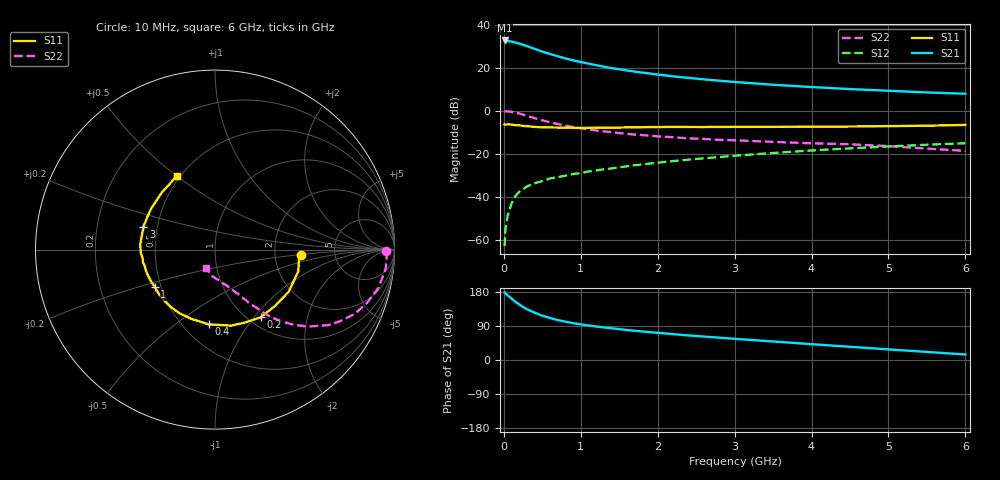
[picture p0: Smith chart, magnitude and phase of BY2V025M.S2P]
! SIEMENS Small Signal Semiconductors
! BFY420
! Si NPN RF SIEGET Grounded Emitter Transistor in MICRO-X
! VCE = 2 V  IC = 25 mA
! Common Emitter S-Parameters:  October  1996
# GHz  S  MA  R  50
!  f  S11  S21  S12  S22
! GHz  MAG  ANG  MAG  ANG  MAG  ANG  MAG  ANG
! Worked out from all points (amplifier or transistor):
!   36 points, 10 MHz to 6 GHz, reference 50 ohm
!   highest |S21| = 32.6 dB at 10 MHz (marker M1)
!   |S21| within 3 dB of that: start of sweep to 327.9 MHz
!   unconditionally stable (mu >= 1): start of sweep to 10.06 MHz; 1.732 GHz to end of sweep
!   at 250 MHz: K = 0.33, MSG = 33.6 dB, |S12| = -36.6 dB
!   at 1.4 GHz: K = 0.95, MSG = 23.4 dB, |S12| = -26.9 dB
!   at 6 GHz: K = 1.07, MAG = 9.9 dB, |S12| = -15.2 dB
!   S11 on the Smith chart (normalised r, x): 10 MHz: 2.82, -0.21; 200 MHz: 1.14, -1.08; 400 MHz: 0.66, -0.67; 1 GHz: 0.46, -0.23; 3 GHz: 0.42, +0.13; 6 GHz: 0.48, +0.50
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0.01  0.4791 -3.4  42.9 178.6  0.0007 119.4  0.9507 -0.5
0.02  0.4714 -6.6  42.76 175.4  0.0017 85.4  0.9582 -2.0
0.1  0.473 -29.8  40.4 162.4  0.0069 79.2  0.9355 -13.2
0.15  0.4587 -43.3  38.34 153.5  0.0102 74.1  0.8978 -19.3
0.2  0.4553 -56.0  36.35 146.8  0.0129 71.5  0.8571 -24.7
0.25  0.4396 -67.4  33.93 139.8  0.0148 67.5  0.8053 -29.6
0.3  0.4334 -77.9  31.62 134.1  0.0172 65.9  0.7588 -33.7
0.4  0.4178 -94.9  27.37 125.0  0.0203 62.6  0.6688 -39.9
0.5  0.4078 -109.0  23.56 116.9  0.023 59.9  0.5955 -44.3
0.6  0.4063 -120.0  20.78 110.9  0.0263 59.4  0.5357 -47.7
0.7  0.4032 -128.8  18.44 105.5  0.0283 59.2  0.4879 -50.4
0.8  0.4012 -136.5  16.4 101.1  0.0305 58.5  0.4471 -52.3
1  0.3944 -148.2  13.47 94.1  0.0352 59.0  0.3893 -55.0
1.1  0.3974 -153.1  12.39 91.2  0.0382 59.4  0.3663 -56.7
1.3  0.4014 -160.9  10.52 85.9  0.0432 59.2  0.3286 -58.6
1.6  0.4079 -170.3  8.589 79.2  0.0505 59.0  0.2876 -61.8
2.2  0.4178 176.3  6.27 68.3  0.0668 57.2  0.2402 -67.5
3  0.4182 162.5  4.641 55.9  0.0889 52.8  0.2039 -73.8
3.5  0.4185 154.4  3.996 48.9  0.1032 49.3  0.1873 -78.1
4.5  0.4259 139.9  3.171 34.9  0.1321 40.9  0.1646 -87.0
5.5  0.4454 124.0  2.646 21.3  0.1607 31.4  0.1306 -103.1
6  0.4641 117.3  2.472 14.5  0.1743 26.6  0.1155 -115.1
